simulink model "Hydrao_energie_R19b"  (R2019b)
settings: Solver=ode23t  StartTime=0  StopTime=1  MaxStep=1e-2  RelTol=1e-3
libraries: fl_lib x27, ee_lib x17, nesl_utility x10, dsparch4 x5, simulink x2, sh_lib x1

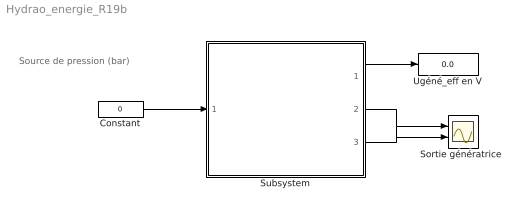
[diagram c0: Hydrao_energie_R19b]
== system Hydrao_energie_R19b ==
  note: Source de pression (bar)
  Constant : Constant  Value=0
  "Sortie génératrice " : Scope  NumInputPorts=2
  Subsystem : Subsystem
  Ugéné_eff en V : Display
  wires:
  Constant/1 -> Subsystem/1(In1)
  Subsystem/1(Uac_eff) -> Ugéné_eff en V/1
  Subsystem/2(Tension inst) -> "Sortie génératrice "/1
  Subsystem/3(Courant inst) -> "Sortie génératrice "/2

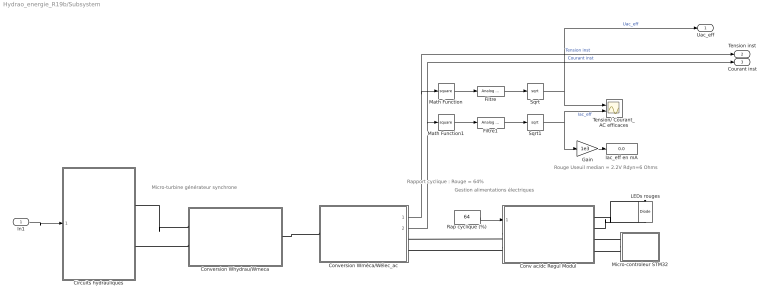
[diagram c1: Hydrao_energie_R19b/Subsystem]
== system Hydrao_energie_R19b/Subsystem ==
  note: Rouge Useuil median = 2.2V Rdyn=6 Ohms
  note: Gestion alimentations électriques
  note: Micro-turbine générateur synchrone
  note: Rapport cyclique : Rouge = 64%
  In1 : Inport
  Circuits hydrauliques : Subsystem
  Conv ac/dc Regul Modul : Subsystem
  Conversion Whydrau/Wmeca : Subsystem
  Conversion Wméca/Wélec_ac : Subsystem
  Filtre : dsparch4/Analog Filter Design  method=Bessel  filttype=Lowpass  N=5  Wlo=50  Whi=80  Rp=2  Rs=40
  Filtre1 : dsparch4/Analog Filter Design  method=Bessel  filttype=Lowpass  N=5  Wlo=50  Whi=80  Rp=2  Rs=40
  Gain : Gain  Gain=1e3
  Iac_eff en mA : Display
  LEDs rouges : ee_lib/Semiconductors & Converters/Diode  ModelType=ee.enum.diode.modelType.pwl  Vf=2.2 V  Ron=6 Ohm  Goff=1e-8 S  prmExp=ee.enum.diode.expParam.useTwo  I12=[0.01, 5] mA  V12=[1.5, 1.85] V  IS=1e-12 A  ec=1  I1=0.0137 A  V1=0.6 V  RS=0 Ohm  Tmeas=25 degC  N_series=1  N_parallel=5  Rz=0.3 Ohm  BV=100 V  C_param=ee.enum.diode.capParam.fixed  CJ=5 pF  CJ0=5 pF  VJ=1 V  Mgrad=0.5  Vvec=[.1, 10, 100] V  Cvec=[3.5, 1, .4] pF  FC=0.5  Q_param=ee.enum.diode.recoveryParam.off  iRM=-7.15 A  iF=4 A  didt=-750 A/us  trr_factor=3  trr=115 ns  Qrr=1500 s*uA  TT=50 ns  tau=100 ns  T_param=ee.enum.diode.temperatureParam.off  IS_T2=1.25e-7 A  I1_T2=0.245 A  V1_T2=0.5 V  Tmeas2=125 degC  EG_param=ee.enum.diode.egapParam.material_si  EG=1.11 eV  XTI_param=ee.enum.diode.xtiParam.pn  XTI=3  dBVdT=0 V/K  Tdevice=25 degC  i_specify=off  i_priority=None  i=0 A  i_nominal_specify=off  i_nominal_unit=A  i_nominal_value=1  v_specify=off  v_priority=None  v=0 V  v_nominal_specify=off  v_nominal_unit=V  v_nominal_value=1  i_capacitor_specify=off  i_capacitor_priority=None  i_capacitor=0 A  i_capacitor_nominal_specify=off  i_capacitor_nominal_unit=A  i_capacitor_nominal_value=1  v_capacitor_specify=off  v_capacitor_priority=None  v_capacitor=0 V  v_capacitor_nominal_specify=off  v_capacitor_nominal_unit=V  v_capacitor_nominal_value=1  power_dissipated_specify=off  power_dissipated_priority=None  power_dissipated=0 W  power_dissipated_nominal_specify=off  power_dissipated_nominal_unit=W  power_dissipated_nominal_value=1  thermal_network_parameterization=ee.enum.thermalNetworkTopology.cauer  Rth=[0, 10] K/W  Rth_Foster=[4, 6] K/W  thermal_mass_parameterization=ee.enum.thermalNetwork.timeconstant  thermal_mass=[0, 1] J/K  thermal_mass_Foster=[1.5, 3] J/K  thermal_time_constant=[0, 10] s  thermal_time_constant_Foster=[6, 18] s  thermal_mass_initial_temperatures=[25, 25] degC
  Math Function : Math  Operator=square  SignedPower=off
  Math Function1 : Math  Operator=square  SignedPower=off
  Micro-controleur STM32 : Subsystem
  Rap cyclique (%) : Constant  Value=64
  Sqrt : Sqrt
  Sqrt1 : Sqrt
  Tension/ Courant_AC efficaces : Scope  NumInputPorts=2
  Uac_eff : Outport
  Tension inst : Outport  Port=2
  Courant inst : Outport  Port=3
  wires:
  Conversion Wméca/Wélec_ac/2(Flux: courant_ac) -> Courant inst/1, Math Function1/1  "Courant inst"
  Math Function/1 -> Filtre/1
  Filtre/1 -> Sqrt/1
  Sqrt/1 -> Uac_eff/1, Tension/ Courant_AC efficaces/1  "Uac_eff"
  Gain/1 -> Iac_eff en mA/1
  Rap cyclique (%)/1 -> Conv ac/dc Regul Modul/1(Modul LEDs)
  Sqrt1/1 -> Tension/ Courant_AC efficaces/2, Gain/1  "Iac_eff"
  Filtre1/1 -> Sqrt1/1
  Conversion Wméca/Wélec_ac/1(" Effort : tension_ac") -> Tension inst/1, Math Function/1  "Tension inst"
  Math Function1/1 -> Filtre1/1
  In1/1 -> Circuits hydrauliques/1(Pression source)
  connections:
  Conv ac/dc Regul Modul/LConn1 -- Conversion Wméca/Wélec_ac/RConn1
  Circuits hydrauliques/RConn2 -- Conversion Whydrau/Wmeca/LConn2
  Micro-controleur STM32/LConn2 -- Conv ac/dc Regul Modul/RConn4
  Conversion Whydrau/Wmeca/RConn1 -- Conversion Wméca/Wélec_ac/LConn1
  LEDs rouges/RConn1 -- Conv ac/dc Regul Modul/RConn2
  Circuits hydrauliques/RConn1 -- Conversion Whydrau/Wmeca/LConn1
  Micro-controleur STM32/LConn1 -- Conv ac/dc Regul Modul/RConn3
  LEDs rouges/LConn1 -- Conv ac/dc Regul Modul/RConn1
  Conv ac/dc Regul Modul/LConn2 -- Conversion Wméca/Wélec_ac/RConn2

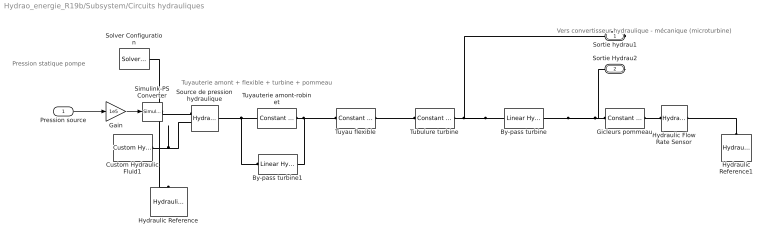
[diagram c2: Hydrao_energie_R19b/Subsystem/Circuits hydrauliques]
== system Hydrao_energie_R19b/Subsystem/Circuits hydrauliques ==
  note: Pression statique pompe
  note: Tuyauterie amont + flexible + turbine + pommeau
  note: Vers convertisseur hydraulique - mécanique (microturbine)
  Pression source : Inport
  By-pass turbine : fl_lib/Hydraulic/Hydraulic Elements/Linear Hydraulic Resistance  Commented=on  resistance=1e0 Pa/(m^3/s)  q_specify=off  q_priority=None  q=0.001 m^3/s  q_nominal_specify=off  q_nominal_unit=m^3/s  q_nominal_value=1  p_specify=off  p_priority=None  p=0 Pa  p_nominal_specify=off  p_nominal_unit=Pa  p_nominal_value=1
  By-pass turbine1 : fl_lib/Hydraulic/Hydraulic Elements/Linear Hydraulic Resistance  Commented=on  resistance=1e0 Pa/(m^3/s)  q_specify=off  q_priority=None  q=0.001 m^3/s  q_nominal_specify=off  q_nominal_unit=m^3/s  q_nominal_value=1  p_specify=off  p_priority=None  p=0 Pa  p_nominal_specify=off  p_nominal_unit=Pa  p_nominal_value=1
  Custom Hydraulic Fluid1 : fl_lib/Hydraulic/Hydraulic Utilities/Custom Hydraulic Fluid  density=994 kg/m^3  viscosity_kin=7.35e-7 m^2/s  bulk=8e8 Pa  alpha=0.005  range_error=2
  Gain : Gain  Gain=1e5
  Gicleurs pommeau : fl_lib/Hydraulic/Hydraulic Elements/Constant Area Hydraulic Orifice  area=20e-6 m^2  C_d=0.4  lam_spec=2  B_lam=0.999  Re_cr=1e0  q_specify=off  q_priority=None  q=0.001 m^3/s  q_nominal_specify=off  q_nominal_unit=m^3/s  q_nominal_value=1  p_specify=off  p_priority=None  p=0 Pa  p_nominal_specify=off  p_nominal_unit=Pa  p_nominal_value=1
  Hydraulic Flow Rate Sensor : fl_lib/Hydraulic/Hydraulic Sensors/Hydraulic Flow Rate Sensor
  Hydraulic Reference : fl_lib/Hydraulic/Hydraulic Elements/Hydraulic Reference
  Hydraulic Reference1 : fl_lib/Hydraulic/Hydraulic Elements/Hydraulic Reference
  Simulink-PS Converter : nesl_utility/Simulink-PS Converter  PhysicalDomain=network_engine_domain  SubClassName=ps_input  LeftPortType=input  RightPortType=output  PseudoPeriodic=off  Frequencies=[]  NoiseDistribution=none  NoiseParameters=[]  Unit=1  AffineConversion=off  FilteringAndDerivatives=provide  SimscapeFilterOrder=1  InputFilterTimeConstant=0.001  UdotUserProvided=0
  Solver Configuration : nesl_utility/Solver Configuration  PhysicalDomain=network_engine_domain  SubClassName=solver  LeftPortType=input  RightPortType=generic  Tones=[]  Harmonics=[]  SimulateNoise=off  Profile=off  UseLocalSampling=off  EnableSwitchedLinearOptims=on  FrequencyDomain=off  UseCCode=off  RelTol=0.001  AbsTol=1e-06  MinStep=1e-09  ToWorkspace=off  RevertToSquareIcSolve=off  NumHomotopyIterations=100  PhasorMode=off  PhasorModeNumHarmonics=1  DoDC=off  ResidualTolerance=1e-9  UseLocalSolver=off  LocalSolverChoice=NE_BACKWARD_EULER_ADVANCER  LocalSolverSampleTime=0.001  DoFixedCost=off  MaxNonlinIter=3  MaxModeIter=2  LinearAlgebra=Sparse  EquationFormulation=NE_TIME_EF  DelaysMemoryBudget=1024  AutomaticFiltering=on  FilteringTimeConstant=0.001  PartitionStorageMethod=AS_NEEDED  PartitionMemoryBudget=1024  PartitionMethod=FAST
  Source de pression hydraulique : fl_lib/Hydraulic/Hydraulic Sources/Hydraulic Pressure Source
  Tubulure turbine : fl_lib/Hydraulic/Hydraulic Elements/Constant Area Hydraulic Orifice  area=12.7e-6 m^2  C_d=0.81  lam_spec=2  B_lam=0.999  Re_cr=1e0  q_specify=off  q_priority=None  q=0.001 m^3/s  q_nominal_specify=off  q_nominal_unit=m^3/s  q_nominal_value=1  p_specify=off  p_priority=None  p=0 Pa  p_nominal_specify=off  p_nominal_unit=Pa  p_nominal_value=1
  Tuyau flexible : fl_lib/Hydraulic/Hydraulic Elements/Constant Area Hydraulic Orifice  area=41e-6 m^2  C_d=0.25  lam_spec=2  B_lam=2000  Re_cr=1e0  q_specify=off  q_priority=None  q=0.001 m^3/s  q_nominal_specify=off  q_nominal_unit=m^3/s  q_nominal_value=1  p_specify=off  p_priority=None  p=0 Pa  p_nominal_specify=off  p_nominal_unit=Pa  p_nominal_value=1
  Tuyauterie amont-robinet : fl_lib/Hydraulic/Hydraulic Elements/Constant Area Hydraulic Orifice  area=113e-6 m^2  C_d=0.134  lam_spec=2  B_lam=0.999  Re_cr=1e0  q_specify=off  q_priority=None  q=0.001 m^3/s  q_nominal_specify=off  q_nominal_unit=m^3/s  q_nominal_value=1  p_specify=off  p_priority=None  p=0 Pa  p_nominal_specify=off  p_nominal_unit=Pa  p_nominal_value=1
  Sortie hydrau1 : PMIOPort  Side=Right
  Sortie Hydrau2 : PMIOPort  Port=2  Side=Right
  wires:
  Gain/1 -> Simulink-PS Converter/1
  Pression source/1 -> Gain/1
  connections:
  Custom Hydraulic Fluid1/RConn1 -- Solver Configuration/RConn1 -- Source de pression hydraulique/RConn2 -- Hydraulic Reference/LConn1
  Simulink-PS Converter/RConn1 -- Source de pression hydraulique/RConn1
  By-pass turbine1/LConn1 -- Tuyauterie amont-robinet/LConn1 -- Source de pression hydraulique/LConn1
  Gicleurs pommeau/RConn1 -- Hydraulic Flow Rate Sensor/LConn1
  Gicleurs pommeau/LConn1 -- By-pass turbine/RConn1 -- Sortie Hydrau2/RConn1
  Tuyau flexible/RConn1 -- Tubulure turbine/LConn1
  Tuyauterie amont-robinet/RConn1 -- By-pass turbine1/RConn1 -- Tuyau flexible/LConn1
  Tubulure turbine/RConn1 -- By-pass turbine/LConn1 -- Sortie hydrau1/RConn1
  Hydraulic Reference1/LConn1 -- Hydraulic Flow Rate Sensor/RConn2

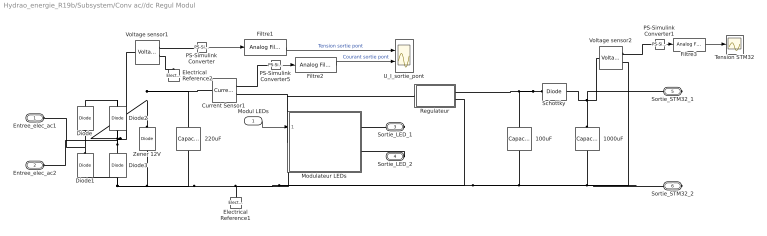
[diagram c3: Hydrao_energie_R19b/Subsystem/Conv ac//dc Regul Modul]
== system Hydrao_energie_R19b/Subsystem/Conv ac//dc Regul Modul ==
  Modul LEDs : Inport
  " 1000uF" : ee_lib/Passive/Capacitor  cap_option=0  c=200 uF  Cvec=[1e-05, 1e-06] F  Vvec=[0, 10] V  CV_table_symmetry=1  f_vec=[1, 10] kHz  DFext_vec=[.8, 1.2]  C_tol=5  enable_C_tol=0  tol_distribution=1  nSigma=4  r=0.1 Ohm  g=0 1/Ohm  averaging_period=0 s  enable_operating_limits=0  operating_limit_action=2  max_working_voltage_range=[-25, 25] V  power_rating=1 W  enable_faults=0  fault_action=1  Cscale_faulted=100  R_faulted=1e-3 Ohm  G_faulted=0 1/Ohm  tau_fault=1e-3 s  enable_temporal_fault=0  t_fault=1 s  enable_behavioral_fault=0  max_permissible_voltage_range=[-100, 100] V  t_fail_on_voltage=1 s  i_specify=off  i_priority=None  i=0 A  i_nominal_specify=off  i_nominal_unit=A  i_nominal_value=1  v_specify=off  v_priority=High  v=3 V  v_nominal_specify=off  v_nominal_unit=V  v_nominal_value=1  vc_specify=on  vc_priority=High  vc=2 V  vc_nominal_specify=off  vc_nominal_unit=V  vc_nominal_value=1
  " 100uF" : ee_lib/Passive/Capacitor  cap_option=0  c=100 uF  Cvec=[1e-05, 1e-06] F  Vvec=[0, 10] V  CV_table_symmetry=1  f_vec=[1, 10] kHz  DFext_vec=[.8, 1.2]  C_tol=5  enable_C_tol=0  tol_distribution=1  nSigma=4  r=0.2 Ohm  g=0 1/Ohm  averaging_period=0 s  enable_operating_limits=0  operating_limit_action=2  max_working_voltage_range=[-25, 25] V  power_rating=1 W  enable_faults=0  fault_action=1  Cscale_faulted=100  R_faulted=1e-3 Ohm  G_faulted=0 1/Ohm  tau_fault=1e-3 s  enable_temporal_fault=0  t_fault=1 s  enable_behavioral_fault=0  max_permissible_voltage_range=[-100, 100] V  t_fail_on_voltage=1 s  i_specify=off  i_priority=None  i=0 A  i_nominal_specify=off  i_nominal_unit=A  i_nominal_value=1  v_specify=off  v_priority=None  v=0 V  v_nominal_specify=off  v_nominal_unit=V  v_nominal_value=1  vc_specify=on  vc_priority=High  vc=3 V  vc_nominal_specify=off  vc_nominal_unit=V  vc_nominal_value=1
  " 220uF" : ee_lib/Passive/Capacitor  cap_option=0  c=220 uF  Cvec=[1e-05, 1e-06] F  Vvec=[0, 10] V  CV_table_symmetry=1  f_vec=[1, 10] kHz  DFext_vec=[.8, 1.2]  C_tol=5  enable_C_tol=0  tol_distribution=1  nSigma=4  r=0.2 Ohm  g=0 1/Ohm  averaging_period=0 s  enable_operating_limits=0  operating_limit_action=2  max_working_voltage_range=[-25, 25] V  power_rating=1 W  enable_faults=0  fault_action=1  Cscale_faulted=100  R_faulted=1e-3 Ohm  G_faulted=0 1/Ohm  tau_fault=1e-3 s  enable_temporal_fault=0  t_fault=1 s  enable_behavioral_fault=0  max_permissible_voltage_range=[-100, 100] V  t_fail_on_voltage=1 s  i_specify=off  i_priority=None  i=0 A  i_nominal_specify=off  i_nominal_unit=A  i_nominal_value=1  v_specify=off  v_priority=None  v=0 V  v_nominal_specify=off  v_nominal_unit=V  v_nominal_value=1  vc_specify=on  vc_priority=High  vc=3 V  vc_nominal_specify=off  vc_nominal_unit=V  vc_nominal_value=1
  Current Sensor1 : fl_lib/Electrical/Electrical Sensors/Current Sensor
  Diode{,1..3} (4 alike) : ee_lib/Semiconductors & Converters/Diode  ModelType=ee.enum.diode.modelType.pwl  Vf=0.4 V  Ron=1 Ohm  Goff=1e-8 S  prmExp=ee.enum.diode.expParam.useTwo  I12=[.0137, .545] A  V12=[.6, .7] V  IS=1e-12 A  ec=1  I1=0.0137 A  V1=0.6 V  RS=0 Ohm  Tmeas=25 degC  N_series=1  N_parallel=1  Rz=0.3 Ohm  BV=100 V  C_param=ee.enum.diode.capParam.fixed  CJ=5 pF  CJ0=5 pF  VJ=1 V  Mgrad=0.5  Vvec=[.1, 10, 100] V  Cvec=[3.5, 1, .4] pF  FC=0.5  Q_param=ee.enum.diode.recoveryParam.off  iRM=-7.15 A  iF=4 A  didt=-750 A/us  trr_factor=3  trr=115 ns  Qrr=1500 s*uA  TT=50 ns  tau=100 ns  T_param=ee.enum.diode.temperatureParam.off  IS_T2=1.25e-7 A  I1_T2=0.245 A  V1_T2=0.5 V  Tmeas2=125 degC  EG_param=ee.enum.diode.egapParam.material_si  EG=1.11 eV  XTI_param=ee.enum.diode.xtiParam.pn  XTI=3  dBVdT=0 V/K  Tdevice=25 degC  i_specify=off  i_priority=None  i=0 A  i_nominal_specify=off  i_nominal_unit=A  i_nominal_value=1  v_specify=off  v_priority=None  v=0 V  v_nominal_specify=off  v_nominal_unit=V  v_nominal_value=1  i_capacitor_specify=off  i_capacitor_priority=None  i_capacitor=0 A  i_capacitor_nominal_specify=off  i_capacitor_nominal_unit=A  i_capacitor_nominal_value=1  v_capacitor_specify=off  v_capacitor_priority=None  v_capacitor=0 V  v_capacitor_nominal_specify=off  v_capacitor_nominal_unit=V  v_capacitor_nominal_value=1  power_dissipated_specify=off  power_dissipated_priority=None  power_dissipated=0 W  power_dissipated_nominal_specify=off  power_dissipated_nominal_unit=W  power_dissipated_nominal_value=1  thermal_network_parameterization=ee.enum.thermalNetworkTopology.cauer  Rth=[0, 10] K/W  Rth_Foster=[4, 6] K/W  thermal_mass_parameterization=ee.enum.thermalNetwork.timeconstant  thermal_mass=[0, 1] J/K  thermal_mass_Foster=[1.5, 3] J/K  thermal_time_constant=[0, 10] s  thermal_time_constant_Foster=[6, 18] s  thermal_mass_initial_temperatures=[25, 25] degC
  Electrical Reference1 : fl_lib/Electrical/Electrical Elements/Electrical Reference
  Electrical Reference2 : fl_lib/Electrical/Electrical Elements/Electrical Reference
  Filtre1 : dsparch4/Analog Filter Design  Commented=through  method=Bessel  filttype=Lowpass  N=3  Wlo=50  Whi=80  Rp=2  Rs=40
  Filtre2 : dsparch4/Analog Filter Design  Commented=through  method=Bessel  filttype=Lowpass  N=3  Wlo=50  Whi=80  Rp=2  Rs=40
  Filtre3 : dsparch4/Analog Filter Design  method=Bessel  filttype=Lowpass  N=3  Wlo=50  Whi=80  Rp=2  Rs=40
  Modulateur LEDs : Subsystem
  PS-Simulink Converter : nesl_utility/PS-Simulink Converter  PhysicalDomain=network_engine_domain  SubClassName=ps_output  LeftPortType=input  RightPortType=output  PseudoPeriodic=off  Frequencies=[]  Unit=V  AffineConversion=off
  PS-Simulink Converter1 : nesl_utility/PS-Simulink Converter  PhysicalDomain=network_engine_domain  SubClassName=ps_output  LeftPortType=input  RightPortType=output  PseudoPeriodic=off  Frequencies=[]  Unit=V  AffineConversion=off
  PS-Simulink Converter5 : nesl_utility/PS-Simulink Converter  PhysicalDomain=network_engine_domain  SubClassName=ps_output  LeftPortType=input  RightPortType=output  PseudoPeriodic=off  Frequencies=[]  Unit=A  AffineConversion=off
  Regulateur : Subsystem
  Schottky : ee_lib/Semiconductors & Converters/Diode  ModelType=ee.enum.diode.modelType.pwl  Vf=0.3 V  Ron=1 Ohm  Goff=1e-8 S  prmExp=ee.enum.diode.expParam.useTwo  I12=[.0137, .545] A  V12=[.6, .7] V  IS=1e-12 A  ec=1  I1=0.0137 A  V1=0.6 V  RS=0 Ohm  Tmeas=25 degC  N_series=1  N_parallel=1  Rz=1 Ohm  BV=100 V  C_param=ee.enum.diode.capParam.fixed  CJ=5 pF  CJ0=5 pF  VJ=1 V  Mgrad=0.5  Vvec=[.1, 10, 100] V  Cvec=[3.5, 1, .4] pF  FC=0.5  Q_param=ee.enum.diode.recoveryParam.off  iRM=-7.15 A  iF=4 A  didt=-750 A/us  trr_factor=3  trr=115 ns  Qrr=1500 s*uA  TT=50 ns  tau=100 ns  T_param=ee.enum.diode.temperatureParam.off  IS_T2=1.25e-7 A  I1_T2=0.245 A  V1_T2=0.5 V  Tmeas2=125 degC  EG_param=ee.enum.diode.egapParam.material_si  EG=1.11 eV  XTI_param=ee.enum.diode.xtiParam.pn  XTI=3  dBVdT=0 V/K  Tdevice=25 degC  i_specify=off  i_priority=None  i=0 A  i_nominal_specify=off  i_nominal_unit=A  i_nominal_value=1  v_specify=off  v_priority=None  v=0 V  v_nominal_specify=off  v_nominal_unit=V  v_nominal_value=1  i_capacitor_specify=off  i_capacitor_priority=None  i_capacitor=0 A  i_capacitor_nominal_specify=off  i_capacitor_nominal_unit=A  i_capacitor_nominal_value=1  v_capacitor_specify=off  v_capacitor_priority=None  v_capacitor=0 V  v_capacitor_nominal_specify=off  v_capacitor_nominal_unit=V  v_capacitor_nominal_value=1  power_dissipated_specify=off  power_dissipated_priority=None  power_dissipated=0 W  power_dissipated_nominal_specify=off  power_dissipated_nominal_unit=W  power_dissipated_nominal_value=1  thermal_network_parameterization=ee.enum.thermalNetworkTopology.cauer  Rth=[0, 10] K/W  Rth_Foster=[4, 6] K/W  thermal_mass_parameterization=ee.enum.thermalNetwork.timeconstant  thermal_mass=[0, 1] J/K  thermal_mass_Foster=[1.5, 3] J/K  thermal_time_constant=[0, 10] s  thermal_time_constant_Foster=[6, 18] s  thermal_mass_initial_temperatures=[25, 25] degC
  Tension STM32 : Scope
  U_I_sortie_pont : Scope  NumInputPorts=2
  Voltage sensor1 : fl_lib/Electrical/Electrical Sensors/Voltage Sensor
  Voltage sensor2 : fl_lib/Electrical/Electrical Sensors/Voltage Sensor
  Zener 12V : ee_lib/Semiconductors & Converters/Diode  ModelType=ee.enum.diode.modelType.pwl  Vf=0.7 V  Ron=0.5 Ohm  Goff=1e-8 S  prmExp=ee.enum.diode.expParam.useTwo  I12=[.0137, .545] A  V12=[.6, .7] V  IS=1e-12 A  ec=1  I1=0.0137 A  V1=0.6 V  RS=0 Ohm  Tmeas=25 degC  N_series=1  N_parallel=1  Rz=5 Ohm  BV=12 V  C_param=ee.enum.diode.capParam.fixed  CJ=5 pF  CJ0=5 pF  VJ=1 V  Mgrad=0.5  Vvec=[.1, 10, 100] V  Cvec=[3.5, 1, .4] pF  FC=0.5  Q_param=ee.enum.diode.recoveryParam.off  iRM=-7.15 A  iF=4 A  didt=-750 A/us  trr_factor=3  trr=115 ns  Qrr=1500 s*uA  TT=50 ns  tau=100 ns  T_param=ee.enum.diode.temperatureParam.off  IS_T2=1.25e-7 A  I1_T2=0.245 A  V1_T2=0.5 V  Tmeas2=125 degC  EG_param=ee.enum.diode.egapParam.material_si  EG=1.11 eV  XTI_param=ee.enum.diode.xtiParam.pn  XTI=3  dBVdT=0 V/K  Tdevice=25 degC  i_specify=off  i_priority=None  i=0 A  i_nominal_specify=off  i_nominal_unit=A  i_nominal_value=1  v_specify=off  v_priority=None  v=0 V  v_nominal_specify=off  v_nominal_unit=V  v_nominal_value=1  i_capacitor_specify=off  i_capacitor_priority=None  i_capacitor=0 A  i_capacitor_nominal_specify=off  i_capacitor_nominal_unit=A  i_capacitor_nominal_value=1  v_capacitor_specify=off  v_capacitor_priority=None  v_capacitor=0 V  v_capacitor_nominal_specify=off  v_capacitor_nominal_unit=V  v_capacitor_nominal_value=1  power_dissipated_specify=off  power_dissipated_priority=None  power_dissipated=0 W  power_dissipated_nominal_specify=off  power_dissipated_nominal_unit=W  power_dissipated_nominal_value=1  thermal_network_parameterization=ee.enum.thermalNetworkTopology.cauer  Rth=[0, 10] K/W  Rth_Foster=[4, 6] K/W  thermal_mass_parameterization=ee.enum.thermalNetwork.timeconstant  thermal_mass=[0, 1] J/K  thermal_mass_Foster=[1.5, 3] J/K  thermal_time_constant=[0, 10] s  thermal_time_constant_Foster=[6, 18] s  thermal_mass_initial_temperatures=[25, 25] degC
  Entree_elec_ac1 : PMIOPort  Side=Left
  Entree_elec_ac2 : PMIOPort  Port=2  Side=Left
  Sortie_LED_1 : PMIOPort  Port=3  Side=Right
  Sortie_LED_2 : PMIOPort  Port=4  Side=Right
  Sortie_STM32_1 : PMIOPort  Port=5  Side=Right
  Sortie_STM32_2 : PMIOPort  Port=6  Side=Right
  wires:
  PS-Simulink Converter1/1 -> Filtre3/1
  Modul LEDs/1 -> Modulateur LEDs/1(Modul LEDs)
  PS-Simulink Converter5/1 -> Filtre2/1
  Filtre1/1 -> U_I_sortie_pont/1  "Tension sortie pont"
  Filtre2/1 -> U_I_sortie_pont/2  "Courant sortie pont"
  PS-Simulink Converter/1 -> Filtre1/1
  Filtre3/1 -> Tension STM32/1
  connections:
  Diode3/LConn1 -- Diode1/LConn1 -- Sortie_STM32_2/RConn1 -- Voltage sensor2/RConn2 -- " 1000uF"/RConn1 -- " 100uF"/RConn1 -- Regulateur/RConn2 -- Modulateur LEDs/LConn2 -- Electrical Reference1/LConn1 -- " 220uF"/RConn1 -- Zener 12V/LConn1
  " 1000uF"/LConn1 -- Schottky/RConn1 -- Voltage sensor2/LConn1 -- Sortie_STM32_1/RConn1
  Diode2/LConn1 -- Entree_elec_ac2/RConn1 -- Diode3/RConn1
  Zener 12V/RConn1 -- " 220uF"/LConn1 -- Current Sensor1/LConn1 -- Diode2/RConn1 -- Diode/RConn1 -- Voltage sensor1/LConn1
  Modulateur LEDs/LConn1 -- Current Sensor1/RConn2 -- Regulateur/LConn1
  Schottky/LConn1 -- Regulateur/RConn1 -- " 100uF"/LConn1
  PS-Simulink Converter/LConn1 -- Voltage sensor1/RConn1
  PS-Simulink Converter5/LConn1 -- Current Sensor1/RConn1
  Voltage sensor1/RConn2 -- Electrical Reference2/LConn1
  PS-Simulink Converter1/LConn1 -- Voltage sensor2/RConn1
  Diode1/RConn1 -- Entree_elec_ac1/RConn1 -- Diode/LConn1
  Modulateur LEDs/RConn1 -- Sortie_LED_1/RConn1
  Sortie_LED_2/RConn1 -- Modulateur LEDs/RConn2

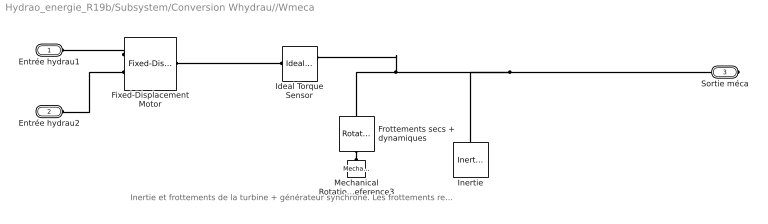
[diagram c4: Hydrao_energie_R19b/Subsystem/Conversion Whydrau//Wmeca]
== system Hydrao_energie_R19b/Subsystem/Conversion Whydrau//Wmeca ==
  note: Inertie et frottements de la turbine + générateur synchrone. Les frottements représentent les pertes mécaniques
  Fixed-Displacement Motor : sh_lib/Pumps and Motors/Fixed-Displacement Motor  D=0.3 cm^3/rad  loss_spec=1  w_nominal=300 rad/s  pr_nominal=100e5 Pa  visc_nominal=1e-6 m^2/s  dens_nominal=997 kg/m^3  efficiency_vol=0.92  no_load_torque=1e-4 N*m  torque_pressure_coeff=1e-7 N*m/Pa  p_diff_eff_TLU=[100000, 1000000, 2000000] Pa  omega_eff_TLU=[25, 50, 100, 200, 300, 400] rad/s  vol_eff_TLU=[.816, .908, .954, .977, .981, .984; .325, .663, .831, .916, .925, .946; .137, .568, .78, .892, .893, .91]  mech_eff_TLU=[.996, .996, .996, .996, .996, .996; .988, .989, .989, .989, .989, .99; .981, .981, .982, .982, .983, .984]  p_diff_loss_TLU=[100000, 1000000, 2000000] Pa  omega_loss_TLU=[25, 50, 100, 200, 300, 400] rad/s  vol_loss_TLU=[.0282, .0253, .0241, .0235, .0291, .0325; .2596, .1271, .1017, .0917, .1216, .1142; .7874, .1901, .141, .1211, .1797, .1978] * 1e-3 m^3/s  mech_loss_TLU=[.002, .002, .002, .002, .002, .002; .06, .055, .055, .055, .055, .05; .19, .19, .18, .18, .17, .16] N*m  pressure_threshold=1e5 Pa  omega_threshold=10 rad/s  quadrant_check=0  pressure_check=0  min_valid_pressure=0 Pa  vol_eff_min=1e-3  vol_eff_max=1  mech_eff_min=1e-3  mech_eff_max=1
  Frottements secs + dynamiques : fl_lib/Mechanical/Rotational Elements/Rotational Friction  brkwy_trq=1.5e-4 N*m  brkwy_vel=0.1 rad/s  Col_trq=1.5e-4 N*m  visc_coef=2.7e-7 N*m/(rad/s)  w_specify=off  w_priority=None  w=0 rad/s  w_nominal_specify=off  w_nominal_unit=rad/s  w_nominal_value=1  t_specify=off  t_priority=None  t=0 N*m  t_nominal_specify=off  t_nominal_unit=N*m  t_nominal_value=1
  Ideal Torque Sensor : fl_lib/Mechanical/Mechanical Sensors/Ideal Torque Sensor
  Inertie : fl_lib/Mechanical/Rotational Elements/Inertia  inertia=1.3e-8 kg*m^2  w_specify=off  w_priority=High  w=0 rad/s  w_nominal_specify=off  w_nominal_unit=rad/s  w_nominal_value=1  t_specify=off  t_priority=None  t=0 N*m  t_nominal_specify=off  t_nominal_unit=N*m  t_nominal_value=1
  Mechanical Rotational Reference3 : fl_lib/Mechanical/Rotational Elements/Mechanical Rotational Reference
  Entrée hydrau1 : PMIOPort  Side=Left
  Entrée hydrau2 : PMIOPort  Port=2  Side=Left
  Sortie méca : PMIOPort  Port=3  Side=Right
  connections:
  Fixed-Displacement Motor/LConn1 -- Entrée hydrau1/RConn1
  Sortie méca/RConn1 -- Frottements secs + dynamiques/LConn1 -- Ideal Torque Sensor/RConn1 -- Inertie/LConn1
  Ideal Torque Sensor/LConn1 -- Fixed-Displacement Motor/RConn1
  Frottements secs + dynamiques/RConn1 -- Mechanical Rotational Reference3/LConn1
  Entrée hydrau2/RConn1 -- Fixed-Displacement Motor/LConn2

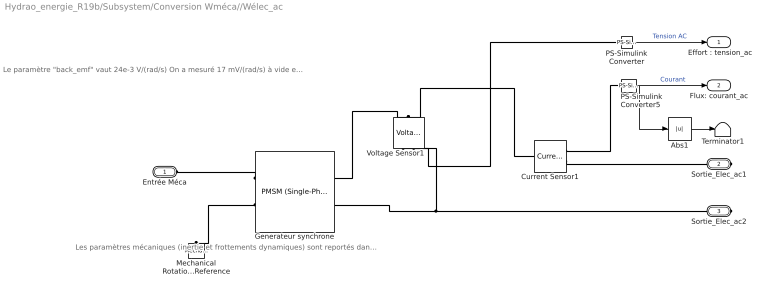
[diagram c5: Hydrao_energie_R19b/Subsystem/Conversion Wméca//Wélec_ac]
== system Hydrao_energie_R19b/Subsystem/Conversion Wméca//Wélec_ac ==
  note: Les paramètres mécaniques (inertie et frottements dynamiques) sont reportés dans le sous-système Conversion Whydrau/Wmeca
  note: Le paramètre "back_emf" vaut 24e-3 V/(rad/s) On a mesuré 17 mV/(rad/s) à vide et on multiplie par racine de 2 car "Back EMF est donnée en valeur max
  " Voltage Sensor1" : fl_lib/Electrical/Electrical Sensors/Voltage Sensor
  Abs1 : Abs
  Current Sensor1 : fl_lib/Electrical/Electrical Sensors/Current Sensor
  Generateur synchrone : ee_lib/Electromechanical/Permanent Magnet/PMSM (Single-Phase)  nPolePairs=1  pmflux_param=2  pm_flux_linkage=0.2 Wb  back_emf_constant=24e-3 V/(rad/s)  L=10 mH  Rs=146 Ohm  J=1e-12 kg*m^2  lam=1e-12 N*m/(rad/s)  pos_standstill=0 deg  i_specify=off  i_priority=High  i=0 A  i_nominal_specify=off  i_nominal_unit=A  i_nominal_value=1  torque_specify=off  torque_priority=None  torque=0 N*m  torque_nominal_specify=off  torque_nominal_unit=N*m  torque_nominal_value=1  angular_velocity_specify=off  angular_velocity_priority=High  angular_velocity=0 rpm  angular_velocity_nominal_specify=off  angular_velocity_nominal_unit=rpm  angular_velocity_nominal_value=1  angular_position_specify=off  angular_position_priority=High  angular_position=0 deg  angular_position_nominal_specify=off  angular_position_nominal_unit=deg  angular_position_nominal_value=1
  Mechanical Rotational Reference : fl_lib/Mechanical/Rotational Elements/Mechanical Rotational Reference
  PS-Simulink Converter : nesl_utility/PS-Simulink Converter  PhysicalDomain=network_engine_domain  SubClassName=ps_output  LeftPortType=input  RightPortType=output  PseudoPeriodic=off  Frequencies=[]  Unit=V  AffineConversion=off
  PS-Simulink Converter5 : nesl_utility/PS-Simulink Converter  PhysicalDomain=network_engine_domain  SubClassName=ps_output  LeftPortType=input  RightPortType=output  PseudoPeriodic=off  Frequencies=[]  Unit=A  AffineConversion=off
  Terminator1 : Terminator
  Entrée Méca : PMIOPort  Side=Left
  Sortie_Elec_ac1 : PMIOPort  Port=2  Side=Right
  Sortie_Elec_ac2 : PMIOPort  Port=3  Side=Right
  " Effort : tension_ac" : Outport  VectorParamsAs1DForOutWhenUnconnected=off
  Flux: courant_ac : Outport  Port=2  VectorParamsAs1DForOutWhenUnconnected=off
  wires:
  PS-Simulink Converter/1 -> " Effort : tension_ac"/1  "Tension AC"
  PS-Simulink Converter5/1 -> Abs1/1, Flux: courant_ac/1  "Courant"
  Abs1/1 -> Terminator1/1
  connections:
  Generateur synchrone/RConn2 -- Mechanical Rotational Reference/LConn1
  Generateur synchrone/RConn1 -- Entrée Méca/RConn1
  " Voltage Sensor1"/LConn1 -- Current Sensor1/LConn1 -- Generateur synchrone/LConn1
  PS-Simulink Converter/LConn1 -- " Voltage Sensor1"/RConn1
  Sortie_Elec_ac2/RConn1 -- " Voltage Sensor1"/RConn2 -- Generateur synchrone/LConn2
  Current Sensor1/RConn2 -- Sortie_Elec_ac1/RConn1
  PS-Simulink Converter5/LConn1 -- Current Sensor1/RConn1

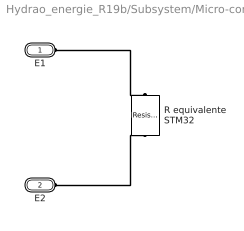
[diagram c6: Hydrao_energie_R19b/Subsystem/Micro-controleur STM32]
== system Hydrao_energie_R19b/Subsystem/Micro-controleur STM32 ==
  R equivalente STM32 : ee_lib/Passive/Resistor  R=10 kOhm  R_tol=5  enable_R_tol=0  tol_distribution=1  nSigma=4  enable_operating_limits=0  operating_limit_action=2  max_working_voltage=100 V  power_rating=1 W  enable_faults=0  fault_action=1  R_faulted=inf Ohm  enable_temporal_fault=0  t_fault=1 s  enable_behavioral_fault=0  max_permissible_current=1 A  t_fail_on_current=1 s  noise_mode=0  sample_time=1e-3 s  repeatability=1  auto_seed=3499211588  user_seed=0  Tdevice=25 degC  alpha=3.93e-3 1/K  Tmeas=25 degC  thermal_mass=100 J/K  power_derating_T1=70 degC  power_derating_T2=155 degC  operating_temperature_range_vec=[-50, 150] degC  temperature_specify=off  temperature_priority=High  temperature=298.15 K  temperature_nominal_specify=off  temperature_nominal_unit=K  temperature_nominal_value=1
  E1 : PMIOPort  Side=Left
  E2 : PMIOPort  Port=2  Side=Left
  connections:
  E2/RConn1 -- R equivalente STM32/RConn1
  E1/RConn1 -- R equivalente STM32/LConn1

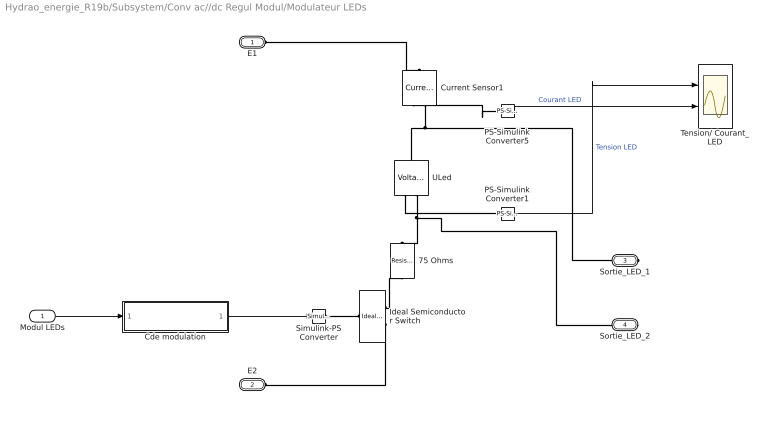
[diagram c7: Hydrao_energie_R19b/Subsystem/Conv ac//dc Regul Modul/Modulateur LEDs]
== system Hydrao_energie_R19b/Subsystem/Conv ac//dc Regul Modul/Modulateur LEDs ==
  Modul LEDs : Inport
  75 Ohms : ee_lib/Passive/Resistor  R=75 Ohm  R_tol=5  enable_R_tol=0  tol_distribution=1  nSigma=4  enable_operating_limits=0  operating_limit_action=2  max_working_voltage=100 V  power_rating=1 W  enable_faults=0  fault_action=1  R_faulted=inf Ohm  enable_temporal_fault=0  t_fault=1 s  enable_behavioral_fault=0  max_permissible_current=1 A  t_fail_on_current=1 s  noise_mode=0  sample_time=1e-3 s  repeatability=1  auto_seed=545404223  user_seed=0  Tdevice=25 degC  alpha=3.93e-3 1/K  Tmeas=25 degC  thermal_mass=100 J/K  power_derating_T1=70 degC  power_derating_T2=155 degC  operating_temperature_range_vec=[-50, 150] degC  temperature_specify=off  temperature_priority=High  temperature=298.15 K  temperature_nominal_specify=off  temperature_nominal_unit=K  temperature_nominal_value=1
  Cde modulation : Subsystem
  Current Sensor1 : fl_lib/Electrical/Electrical Sensors/Current Sensor
  Ideal Semiconductor Switch : ee_lib/Semiconductors & Converters/Ideal Semiconductor Switch  Ron=0.1 Ohm  Goff=1e-6 1/Ohm  Vth=0.5 V  diode_param=3  diode_Vf=0.8 V  diode_Ron=0.001 Ohm  diode_Goff=1e-5 1/Ohm  diode_C=50e-9 F  diode_iRM=-235 A  diode_iF=300 A  diode_idot=-50 A/us  diode_trr_param=1  diode_trr_factor=3  diode_trr=15 us  diode_Qrr=1500 s*uA
  PS-Simulink Converter1 : nesl_utility/PS-Simulink Converter  PhysicalDomain=network_engine_domain  SubClassName=ps_output  LeftPortType=input  RightPortType=output  PseudoPeriodic=off  Frequencies=[]  Unit=V  AffineConversion=off
  PS-Simulink Converter5 : nesl_utility/PS-Simulink Converter  PhysicalDomain=network_engine_domain  SubClassName=ps_output  LeftPortType=input  RightPortType=output  PseudoPeriodic=off  Frequencies=[]  Unit=A  AffineConversion=off
  Simulink-PS Converter : nesl_utility/Simulink-PS Converter  PhysicalDomain=network_engine_domain  SubClassName=ps_input  LeftPortType=input  RightPortType=output  PseudoPeriodic=off  Frequencies=[]  NoiseDistribution=none  NoiseParameters=[]  Unit=1  AffineConversion=off  FilteringAndDerivatives=provide  SimscapeFilterOrder=1  InputFilterTimeConstant=0.001  UdotUserProvided=0
  Tension/ Courant_LED : Scope  NumInputPorts=2
  ULed : fl_lib/Electrical/Electrical Sensors/Voltage Sensor
  E1 : PMIOPort  Side=Left
  E2 : PMIOPort  Port=2  Side=Left
  Sortie_LED_1 : PMIOPort  Port=3  Side=Right
  Sortie_LED_2 : PMIOPort  Port=4  Side=Right
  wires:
  PS-Simulink Converter1/1 -> Tension/ Courant_LED/1  "Tension LED"
  PS-Simulink Converter5/1 -> Tension/ Courant_LED/2  "Courant LED"
  Modul LEDs/1 -> Cde modulation/1(Modul LEDs)
  Cde modulation/1(Out1) -> Simulink-PS Converter/1
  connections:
  ULed/RConn2 -- Sortie_LED_2/RConn1 -- 75 Ohms/LConn1
  E1/RConn1 -- Current Sensor1/LConn1
  Ideal Semiconductor Switch/RConn2 -- E2/RConn1
  Simulink-PS Converter/RConn1 -- Ideal Semiconductor Switch/LConn1
  Ideal Semiconductor Switch/RConn1 -- 75 Ohms/RConn1
  Current Sensor1/RConn2 -- ULed/LConn1 -- Sortie_LED_1/RConn1
  PS-Simulink Converter5/LConn1 -- Current Sensor1/RConn1
  ULed/RConn1 -- PS-Simulink Converter1/LConn1

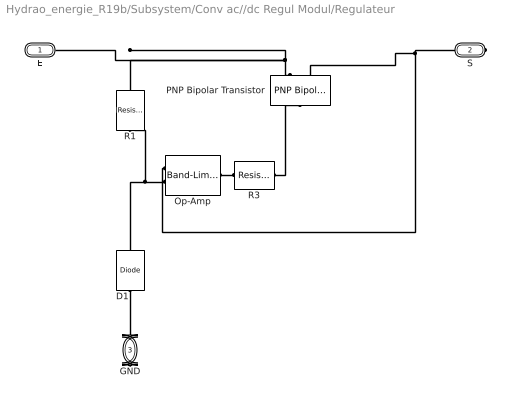
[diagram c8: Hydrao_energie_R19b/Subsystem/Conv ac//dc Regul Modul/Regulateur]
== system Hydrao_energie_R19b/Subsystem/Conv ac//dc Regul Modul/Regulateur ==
  D1 : ee_lib/Semiconductors & Converters/Diode  ModelType=ee.enum.diode.modelType.pwl  Vf=0.6 V  Ron=10 Ohm  Goff=1e-08 S  prmExp=ee.enum.diode.expParam.useTwo  I12="[  0.07 1.5 ] A"  V12="[  0.7 0.8 ] V"  IS=1e-14 A  ec=1  I1=0.0137 A  V1=0.6 V  RS=0.01 Ohm  Tmeas=25 degC  N_series=1  N_parallel=1  Rz=1 Ohm  BV=3.3 V  C_param=ee.enum.diode.capParam.fixed  CJ=5 pF  CJ0=5 pF  VJ=1 V  Mgrad=0.5  Vvec="[  0.1 10 100 ] V"  Cvec="[  3.5 1 0.4 ] pF"  FC=0.5  Q_param=ee.enum.diode.recoveryParam.off  iRM=-7.15 A  iF=4 A  didt=-750 A/us  trr_factor=3  trr=115 ns  Qrr=1500 s*uA  TT=50 ns  tau=100 ns  T_param=ee.enum.diode.temperatureParam.off  IS_T2=1.25e-7 A  I1_T2=0.245 A  V1_T2=0.5 V  Tmeas2=125 degC  EG_param=ee.enum.diode.egapParam.material_si  EG=1.11 eV  XTI_param=ee.enum.diode.xtiParam.pn  XTI=3  dBVdT=0 V/K  Tdevice=25 degC  i_specify=off  i_priority=None  i=0 A  i_nominal_specify=off  i_nominal_unit=A  i_nominal_value=1  v_specify=off  v_priority=None  v=0 V  v_nominal_specify=off  v_nominal_unit=V  v_nominal_value=1  i_capacitor_specify=off  i_capacitor_priority=High  i_capacitor=0 A  i_capacitor_nominal_specify=off  i_capacitor_nominal_unit=A  i_capacitor_nominal_value=1  v_capacitor_specify=off  v_capacitor_priority=None  v_capacitor=0 V  v_capacitor_nominal_specify=off  v_capacitor_nominal_unit=V  v_capacitor_nominal_value=1  power_dissipated_specify=off  power_dissipated_priority=None  power_dissipated=0 W  power_dissipated_nominal_specify=off  power_dissipated_nominal_unit=W  power_dissipated_nominal_value=1  thermal_network_parameterization=ee.enum.thermalNetworkTopology.cauer  Rth=[0, 10] K/W  Rth_Foster=[4, 6] K/W  thermal_mass_parameterization=ee.enum.thermalNetwork.timeconstant  thermal_mass=[0, 1] J/K  thermal_mass_Foster=[1.5, 3] J/K  thermal_time_constant=[0, 10] s  thermal_time_constant_Foster=[6, 18] s  thermal_mass_initial_temperatures=[25, 25] degC
  Op-Amp : ee_lib/Integrated Circuits/Band-Limited Op-Amp  A=100000  Rin=2 MOhm  Rout=100 Ohm  Vmin=-0.5 V  Vmax=30 V  Vdotmax=1e6 V/s  f=2 MHz  V0=0 V
  PNP Bipolar Transistor : ee_lib/Semiconductors & Converters/PNP Bipolar Transistor  parameterization=2  prmDatasheet=1  prmEquCoeff=1  BF=1000  IS=1e-14 A  VAF=200 V  hfe=1000  hoe=50e-7 1/Ohm  Ic_h=-1 A  Vce_h=-15 V  V1=-0.55 V  I1=-1 mA  BR=0.1  Tmeas=25 degC  RC=0.1 Ohm  RE=1e-4 Ohm  RB=1 Ohm  C_BC=5 pF  C_BE=5 pF  TF=0 us  TR=0 us  hfe_T2=125  XTB=0  V1_T2=-0.45 V  I1_T2=-0.5 mA  Tmeas2=125 degC  EG=1.11 eV  XTI=3  ec=1  TdeviceDatasheet=25 degC  TdeviceEquCoeff=25 degC  thermal_network_parameterization=ee.enum.thermalNetworkTopology.cauer  Rth=[0, 10] K/W  Rth_Foster=[4, 6] K/W  thermal_mass_parameterization=ee.enum.thermalNetwork.timeconstant  thermal_mass=[0, 1] J/K  thermal_mass_Foster=[1.5, 3] J/K  thermal_time_constant=[0, 10] s  thermal_time_constant_Foster=[6, 18] s  thermal_mass_initial_temperatures=[25, 25] degC
  R1 : fl_lib/Electrical/Electrical Elements/Resistor  R=1 kOhm  i_specify=off  i_priority=High  i=0 A  i_nominal_specify=off  i_nominal_unit=A  i_nominal_value=1  v_specify=off  v_priority=High  v=0 V  v_nominal_specify=off  v_nominal_unit=V  v_nominal_value=1
  R3 : fl_lib/Electrical/Electrical Elements/Resistor  R=10 kOhm  i_specify=off  i_priority=High  i=0 A  i_nominal_specify=off  i_nominal_unit=A  i_nominal_value=1  v_specify=off  v_priority=High  v=0 V  v_nominal_specify=off  v_nominal_unit=V  v_nominal_value=1
  E : PMIOPort  Side=Left
  S : PMIOPort  Port=2  Side=Right
  GND : PMIOPort  Port=3  Side=Right
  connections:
  R3/RConn1 -- PNP Bipolar Transistor/LConn1
  Op-Amp/LConn2 -- D1/RConn1 -- R1/RConn1
  Op-Amp/RConn1 -- R3/LConn1
  PNP Bipolar Transistor/RConn1 -- R1/LConn1 -- E/RConn1
  Op-Amp/LConn1 -- PNP Bipolar Transistor/RConn2 -- S/RConn1
  D1/LConn1 -- GND/RConn1

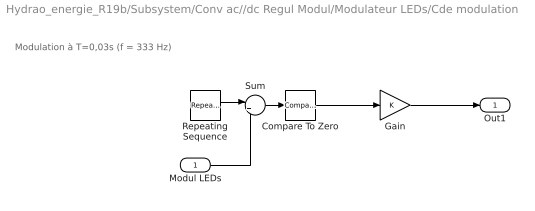
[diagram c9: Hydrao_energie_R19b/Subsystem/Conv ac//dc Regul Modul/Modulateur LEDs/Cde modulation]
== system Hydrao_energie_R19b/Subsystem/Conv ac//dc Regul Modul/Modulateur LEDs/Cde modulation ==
  note: Modulation à T=0,03s (f = 333 Hz)
  Modul LEDs : Inport
  Compare To Zero : simulink/Logic and Bit Operations/Compare To Zero  relop=<  OutDataTypeStr=boolean
  Gain : Gain  OutDataTypeStr=double
  Repeating Sequence : simulink/Sources/Repeating Sequence  rep_seq_t=[0 0.003]  rep_seq_y=[0 100]
  Sum : Sum  Inputs=|+-
  Out1 : Outport  VectorParamsAs1DForOutWhenUnconnected=off
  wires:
  Repeating Sequence/1 -> Sum/1
  Sum/1 -> Compare To Zero/1
  Compare To Zero/1 -> Gain/1
  Modul LEDs/1 -> Sum/2
  Gain/1 -> Out1/1
